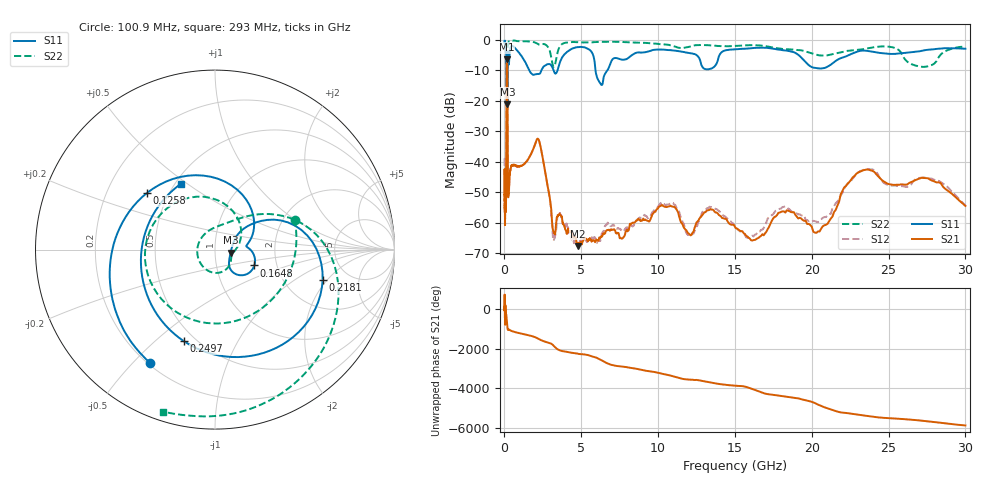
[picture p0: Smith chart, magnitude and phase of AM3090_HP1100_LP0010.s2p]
! Date/Time: Thu, Feb 28, 2019 2:06 PM
! Network Analyzer: Agilent Technologies E8364B Rev: A.07.50.67
! Sweep from 0.010 to 30.000 GHz, 1601 Points, Sweep Type: LOG
! Power Supply: 5.023 V, 0.002 A
# Hz S DB R 50
!freq MagS11 AngS11 MagS21 AngS21 MagS12 AngS12 MagS22 AngS22
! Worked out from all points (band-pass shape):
!   1601 points, 10 MHz to 30 GHz, reference 50 ohm
!   highest |S21| = -6.38 dB at 161.5 MHz (marker M1); lowest = -67.6 dB at 4.781 GHz (marker M2)
!   |S21| within 3 dB of the highest: 140.3 MHz to 188.7 MHz (48.45 MHz wide, 29.5 % of centre)
!   lowest |S11| = -21.1 dB at 190.6 MHz (marker M3), VSWR 1.19, Z = 59.5 - j2.01 ohm
!   |S11| at or under -10 dB: 1.619 GHz to 2.399 GHz (780.5 MHz wide, 38.9 % of centre); 3.2 GHz to 3.454 GHz (254.1 MHz wide, 7.64 % of centre); 5.926 GHz to 6.696 GHz (770.2 MHz wide, 12.2 % of centre)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
!   |S22| runs from -20.2 to -0.2 dB; largest |S21 - S12| = 0.014
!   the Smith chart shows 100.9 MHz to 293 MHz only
!   S11 on the Smith chart (normalised r, x): 100.9 MHz: 0.21, -0.56; 125.8 MHz: 0.38, +0.32; 164.8 MHz: 1.53, -0.29; 218.1 MHz: 3.24, -1.79; 249.7 MHz: 0.43, -0.62; 293 MHz: 0.53, +0.47
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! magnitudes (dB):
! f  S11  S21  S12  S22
! 10 MHz  -0.3  -52.7  -39.0  -0.5
! 38.04 MHz  -0.4  -58.7  -56.3  -1.2
! 48.37 MHz  -0.6  -48.4  -47.1  -1.3
! 100.9 MHz  -2.8  -55.7  -53.7  -6.5
! 125.8 MHz  -6.1  -25.0  -24.9  -8.2
! 144.7 MHz  -14.5  -7.7  -7.7  -18.9
! 161.5 MHz  -12.8  -6.4  -6.4  -17.8
! 164.8 MHz  -12.5  -6.4  -6.4  -17.7
! 190.6 MHz  -21.1  -10.1  -10.1  -15.9
! 218.1 MHz  -4.1  -45.2  -44.8  -2.5
! 249.7 MHz  -5.4  -51.3  -49.5  -0.9
! 293 MHz  -7.7  -49.0  -50.2  -0.5
! 550.5 MHz  -2.1  -41.1  -41.1  -0.2
! 2.084 GHz  -11.2  -32.9  -32.9  -1.0
! 3.22 GHz  -10.3  -63.3  -65.6  -8.9
! 4.781 GHz  -2.3  -67.6  -67.4  -0.7
! 6.234 GHz  -14.2  -64.9  -65.9  -0.6
! 7.926 GHz  -6.3  -62.6  -61.5  -0.7
! 10.49 GHz  -3.2  -54.7  -54.1  -1.4
! 20.51 GHz  -9.3  -62.8  -59.3  -5.1
! 23.48 GHz  -3.5  -42.6  -42.4  -2.9
! 30 GHz  -2.9  -54.4  -54.3  -2.2
